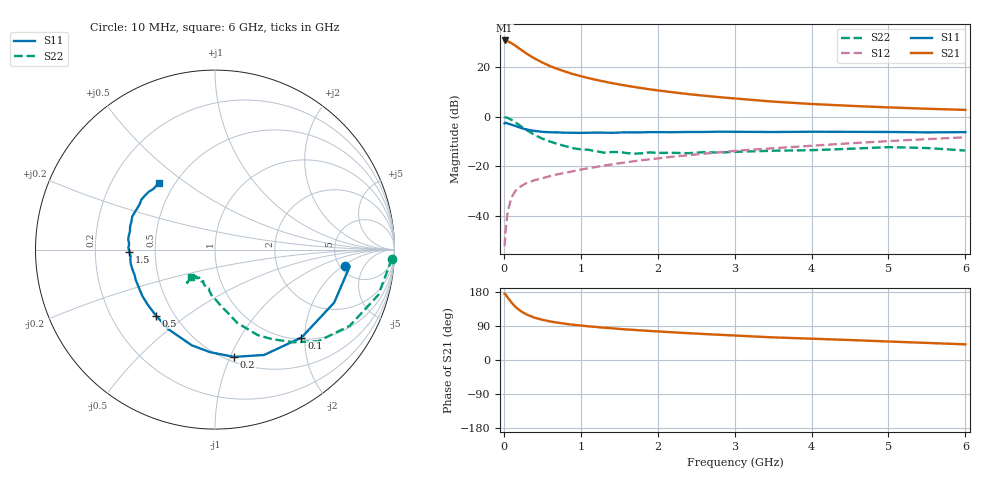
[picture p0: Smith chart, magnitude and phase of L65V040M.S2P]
!  INFINEON TECHNOLOGIES Small Signal Semiconductors
! BFR380L3 , Si-NPN RF-Transistor in TSLP-3-1
!  Vce=5 V,  Ic=40 mA
! Common Emitter S-Parameters:  07. March 2005
#  GHz  S  MA  R  50
! f  S11  S21  S12  S22
! GHz  Mag  Ang  Mag  Ang  Mag  Ang  Mag  Ang
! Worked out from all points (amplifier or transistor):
!   36 points, 10 MHz to 6 GHz, reference 50 ohm
!   highest |S21| = 30.8 dB at 10 MHz (marker M1)
!   |S21| within 3 dB of that: start of sweep to 189.6 MHz
!   unconditionally stable (mu >= 1): 1.944 GHz to 4.789 GHz
!   at 250 MHz: K = 0.39, MSG = 27.1 dB, |S12| = -27.6 dB
!   at 1.4 GHz: K = 0.95, MSG = 16.5 dB, |S12| = -19.3 dB
!   at 6 GHz: K = 0.97, MSG = 5.5 dB, |S12| = -8.3 dB
!   S11 on the Smith chart (normalised r, x): 10 MHz: 5.57, -2.21; 100 MHz: 1.04, -1.93; 200 MHz: 0.55, -1.03; 500 MHz: 0.40, -0.39; 1.5 GHz: 0.35, -0.01; 6 GHz: 0.41, +0.40
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0.01  0.7323 -7.2  34.82 174.9  0.0024 78.3  0.9861 -2.9
0.02  0.7565 -7.1  34.57 173.9  0.0045 83.4  0.9714 -6.2
0.05  0.7267 -24.0  33.59 164.8  0.0121 79.6  0.9444 -15.5
0.1  0.6873 -45.5  30.65 151.6  0.0233 70.8  0.8624 -29.5
0.15  0.6476 -65.0  27.32 140.5  0.0314 63.4  0.7696 -41.5
0.2  0.607 -80.0  23.99 131.9  0.0369 59.3  0.6781 -49.6
0.25  0.5726 -92.6  21.14 125.3  0.0416 55.7  0.5916 -57.5
0.3  0.5485 -103.7  18.65 119.7  0.0457 54.8  0.5319 -63.5
0.4  0.5143 -120.2  15.04 111.7  0.0518 53.2  0.4269 -73.1
0.5  0.4933 -131.9  12.48 106.2  0.0567 53.4  0.3593 -78.5
0.6  0.4842 -141.1  10.57 101.8  0.0627 54.4  0.3146 -84.1
0.7  0.4799 -147.6  9.21 98.5  0.0683 56.1  0.2789 -89.2
0.9  0.4727 -159.6  7.269 93.1  0.0787 58.4  0.2297 -98.1
1.1  0.4733 -166.7  6.028 88.9  0.0908 60.6  0.214 -103.7
1.5  0.4776 -178.6  4.487 82.0  0.1141 62.6  0.1928 -113.9
1.8  0.4823 174.8  3.765 77.9  0.1319 63.4  0.182 -119.5
2.2  0.4847 167.8  3.109 73.0  0.1554 63.9  0.1853 -123.3
2.8  0.4963 158.4  2.484 66.6  0.19 64.3  0.1875 -130.6
3.5  0.4897 149.4  2.016 59.7  0.2295 62.8  0.2047 -130.2
4.5  0.4936 143.0  1.658 52.7  0.2894 61.7  0.2242 -130.4
5.5  0.4813 135.1  1.446 45.1  0.3513 58.2  0.232 -130.1
6  0.4865 129.9  1.371 41.3  0.3833 56.2  0.2064 -131.3
